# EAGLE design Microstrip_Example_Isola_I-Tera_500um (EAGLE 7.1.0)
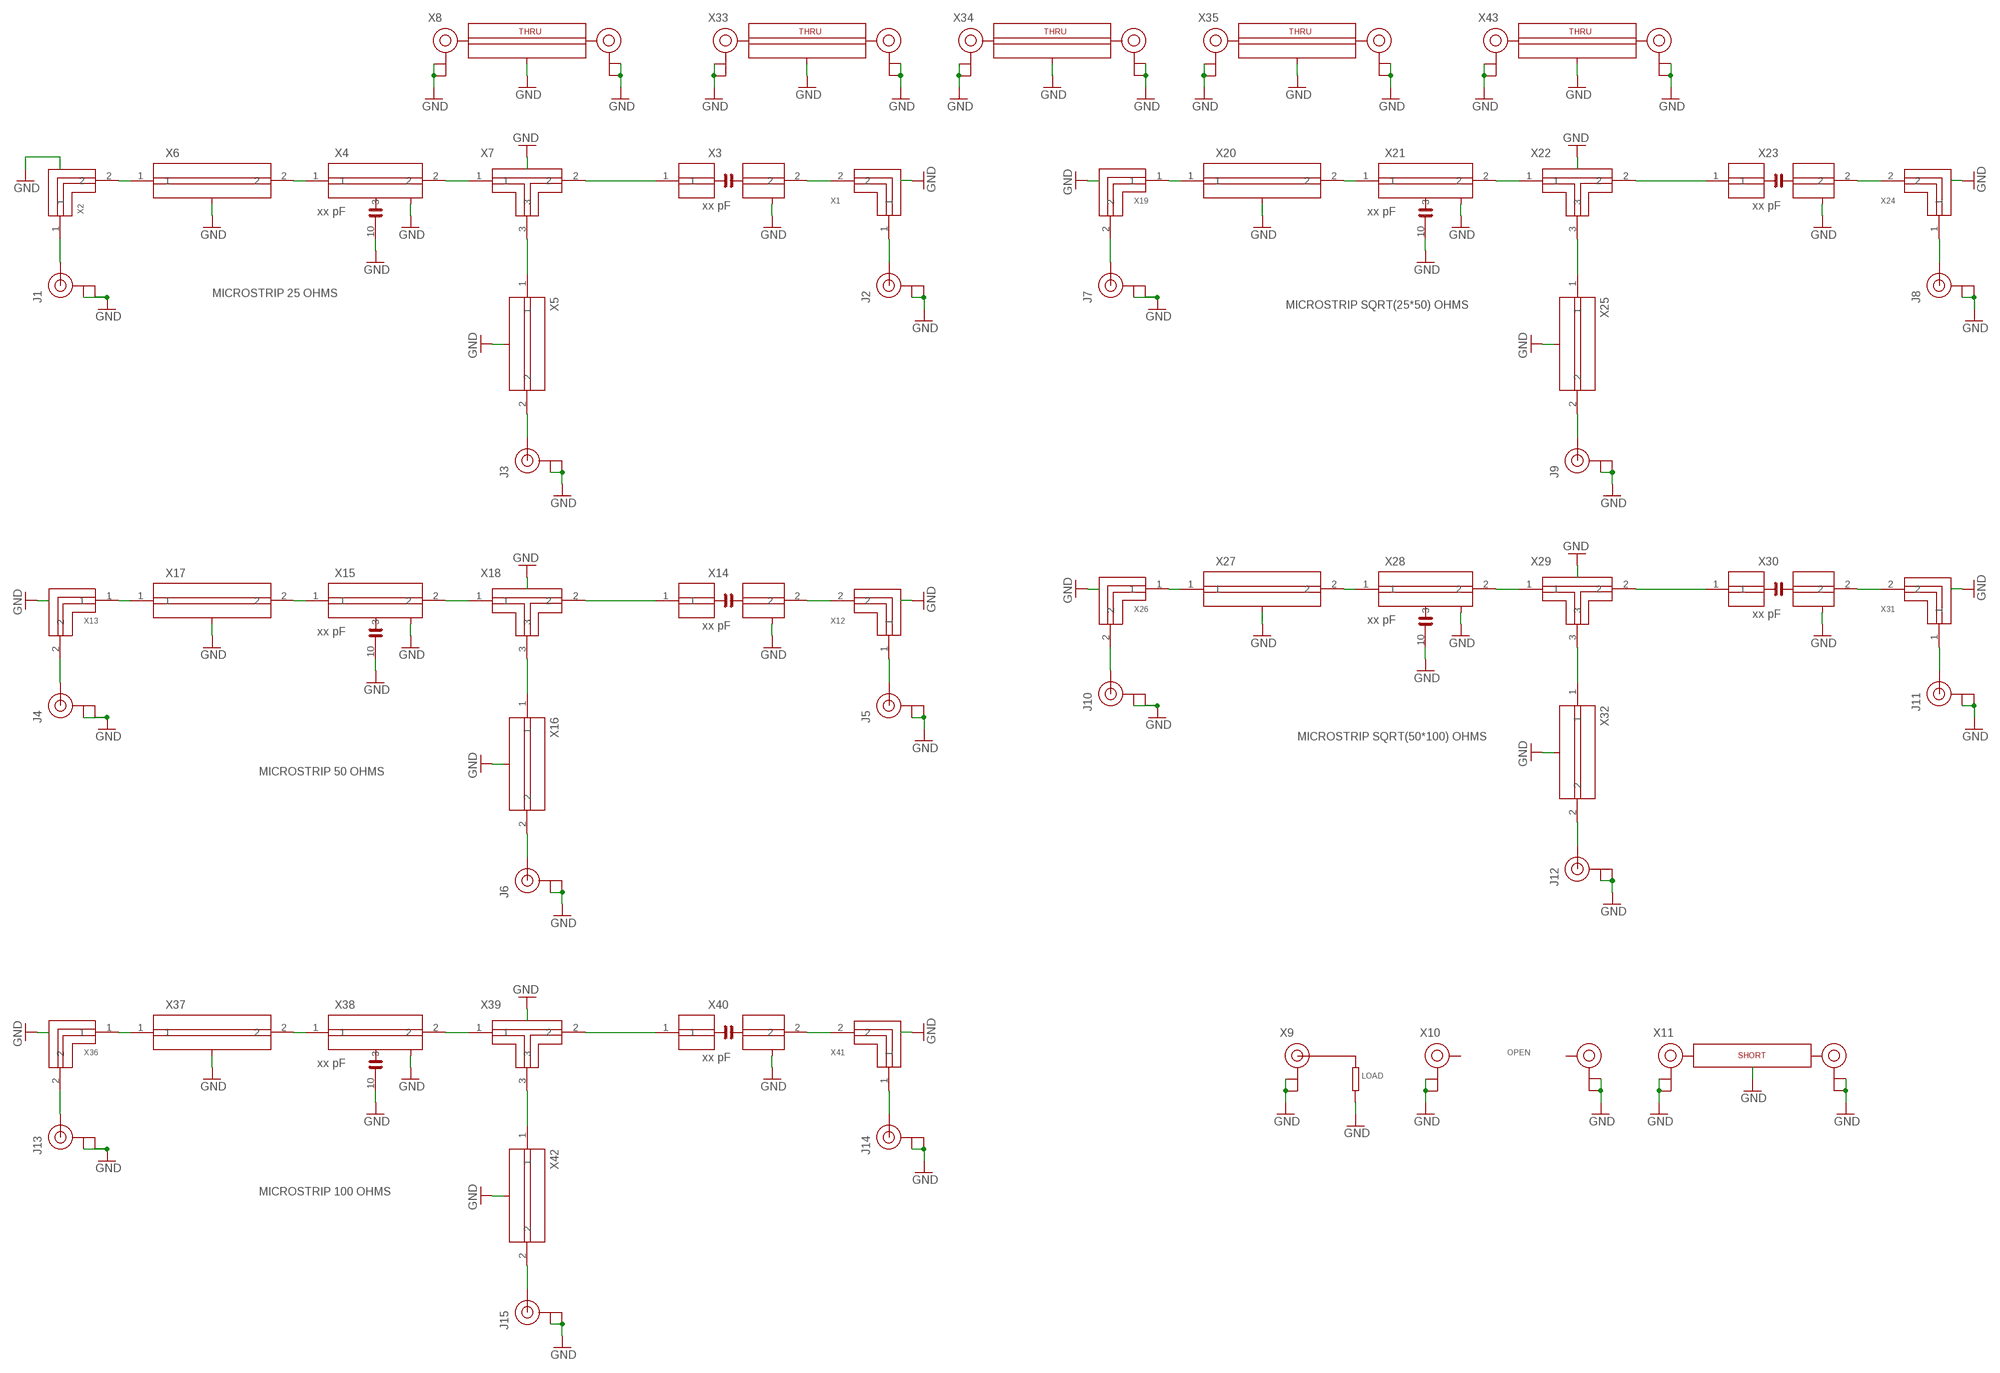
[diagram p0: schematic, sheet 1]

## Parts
J1  U.FL  [U.FL]
J2  U.FL  [U.FL]
J3  U.FL  [U.FL]
J4  U.FL  [U.FL]
J5  U.FL  [U.FL]
J6  U.FL  [U.FL]
J7  U.FL  [U.FL]
J8  U.FL  [U.FL]
J9  U.FL  [U.FL]
J10  U.FL  [U.FL]
J11  U.FL  [U.FL]
J12  U.FL  [U.FL]
J13  U.FL  [U.FL]
J14  U.FL  [U.FL]
J15  U.FL  [U.FL]
X1  CHIPDESIGN_MICROSTRIP_25_OHM_L  [MICROSTRIP_25_OHM_LEFT]
X2  CHIPDESIGN_MICROSTRIP_25_OHM_R  [MICROSTRIP_25_OHM_RIGHT]
X3  xx pF  CHIPDESIGN_MICROSTRIP_25_OHM_SERIES_0402  [MICROSTRIP_25_OHM_0402_SERIES]
X4  xx pF  CHIPDESIGN_MICROSTRIP_25_OHM_SHUNT_0402  [MICROSTRIP_25_OHM_0402_SHUNT]
X5  CHIPDESIGN_MICROSTRIP_25_OHM_TLINE_SHORT  [MICROSTRIP_25_OHM_TLINE_SHORT]
X6  CHIPDESIGN_MICROSTRIP_25_OHM_TLINE_LONG  [MICROSTRIP_25_OHM_TLINE_LONG]
X7  CHIPDESIGN_MICROSTRIP_25_OHM_TJUNCTION  [MICROSTRIP_25_OHM_TEE]
X8  CHIPDESIGN_MICROSTRIP_25_OHM_THRU  [MICROSTRIP_25_OHM_THRU]
X9  LOAD_MICROSTRIP  [LOAD_MICROSTRIP]
X10  OPEN  [OPEN]
X11  SHORT  [SHORT]
X12  CHIPDESIGN_MICROSTRIP_50_OHM_L  [MICROSTRIP_50_OHM_LEFT]
X13  CHIPDESIGN_MICROSTRIP_50_OHM_R  [MICROSTRIP_50_OHM_RIGHT]
X14  xx pF  CHIPDESIGN_MICROSTRIP_50_OHM_SERIES_0402  [MICROSTRIP_50_OHM_0402_SERIES]
X15  xx pF  CHIPDESIGN_MICROSTRIP_50_OHM_SHUNT_0402  [MICROSTRIP_50_OHM_0402_SHUNT]
X16  CHIPDESIGN_MICROSTRIP_50_OHM_TLINE_SHORT  [MICROSTRIP_50_OHM_TLINE_SHORT]
X17  CHIPDESIGN_MICROSTRIP_50_OHM_TLINE_LONG  [MICROSTRIP_50_OHM_TLINE_LONG]
X18  CHIPDESIGN_MICROSTRIP_50_OHM_TJUNCTION  [MICROSTRIP_50_OHM_TEE]
X19  CHIPDESIGN_MICROSTRIP_35_OHM_R  [MICROSTRIP_35_OHM_RIGHT]
X20  CHIPDESIGN_MICROSTRIP_35_OHM_TLINE_LONG  [MICROSTRIP_35_OHM_TLINE_LONG]
X21  xx pF  CHIPDESIGN_MICROSTRIP_35_OHM_SHUNT_0402  [MICROSTRIP_35_OHM_0402_SHUNT]
X22  CHIPDESIGN_MICROSTRIP_35_OHM_TJUNCTION  [MICROSTRIP_35_OHM_TEE]
X23  xx pF  CHIPDESIGN_MICROSTRIP_35_OHM_SERIES_0402  [MICROSTRIP_35_OHM_0402_SERIES]
X24  CHIPDESIGN_MICROSTRIP_35_OHM_L  [MICROSTRIP_35_OHM_LEFT]
X25  CHIPDESIGN_MICROSTRIP_35_OHM_TLINE_SHORT  [MICROSTRIP_35_OHM_TLINE_SHORT]
X26  CHIPDESIGN_MICROSTRIP_70_OHM_R  [MICROSTRIP_70_OHM_RIGHT]
X27  CHIPDESIGN_MICROSTRIP_70_OHM_TLINE_LONG  [MICROSTRIP_70_OHM_TLINE_LONG]
X28  xx pF  CHIPDESIGN_MICROSTRIP_70_OHM_SHUNT_0402  [MICROSTRIP_70_OHM_0402_SHUNT]
X29  CHIPDESIGN_MICROSTRIP_70_OHM_TJUNCTION  [MICROSTRIP_70_OHM_TEE]
X30  xx pF  CHIPDESIGN_MICROSTRIP_70_OHM_SERIES_0402  [MICROSTRIP_70_OHM_0402_SERIES]
X31  CHIPDESIGN_MICROSTRIP_70_OHM_L  [MICROSTRIP_70_OHM_LEFT]
X32  CHIPDESIGN_MICROSTRIP_70_OHM_TLINE_SHORT  [MICROSTRIP_70_OHM_TLINE_SHORT]
X33  CHIPDESIGN_MICROSTRIP_35_OHM_THRU  [MICROSTRIP_35_OHM_THRU]
X34  CHIPDESIGN_MICROSTRIP_50_OHM_THRU  [MICROSTRIP_50_OHM_THRU]
X35  CHIPDESIGN_MICROSTRIP_70_OHM_THRU  [MICROSTRIP_70_OHM_THRU]
X36  CHIPDESIGN_MICROSTRIP_100_OHM_R  [MICROSTRIP_100_OHM_RIGHT]
X37  CHIPDESIGN_MICROSTRIP_100_OHM_TLINE_LONG  [MICROSTRIP_100_OHM_TLINE_LONG]
X38  xx pF  CHIPDESIGN_MICROSTRIP_100_OHM_SHUNT_0402  [MICROSTRIP_100_OHM_0402_SHUNT]
X39  CHIPDESIGN_MICROSTRIP_100_OHM_TJUNCTION  [MICROSTRIP_100_OHM_TEE]
X40  xx pF  CHIPDESIGN_MICROSTRIP_100_OHM_SERIES_0402  [MICROSTRIP_100_OHM_0402_SERIES]
X41  CHIPDESIGN_MICROSTRIP_100_OHM_L  [MICROSTRIP_100_OHM_LEFT]
X42  CHIPDESIGN_MICROSTRIP_100_OHM_TLINE_SHORT  [MICROSTRIP_100_OHM_TLINE_SHORT]
X43  CHIPDESIGN_MICROSTRIP_100_OHM_THRU  [MICROSTRIP_100_OHM_THRU]

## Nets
GND: J1.P$1(GND) J1.P$2(GND) J2.P$1(GND) J2.P$2(GND) J3.P$1(GND) J3.P$2(GND) J4.P$1(GND) J4.P$2(GND) J5.P$1(GND) J5.P$2(GND) J6.P$1(GND) J6.P$2(GND) J7.P$1(GND) J7.P$2(GND) J8.P$1(GND) J8.P$2(GND) J9.P$1(GND) J9.P$2(GND) J10.P$1(GND) J10.P$2(GND) J11.P$1(GND) J11.P$2(GND) J12.P$1(GND) J12.P$2(GND) J13.P$1(GND) J13.P$2(GND) J14.P$1(GND) J14.P$2(GND) J15.P$1(GND) J15.P$2(GND) X1.P$1(GND) X1.P$2(GND) X1.P$3(GND) X1.P$4(GND) X1.P$5(GND) X1.P$6(GND) X1.P$7(GND) X1.P$8(GND) X2.P$1(GND) X2.P$2(GND) X2.P$3(GND) X2.P$4(GND) X2.P$5(GND) X2.P$6(GND) X2.P$7(GND) X2.P$8(GND) X3.P$2(GND) X3.P$3(GND) X3.P$4(GND) X3.P$5(GND) X3.P$6(GND) X3.P$7(GND) X3.P$8(GND) X3.P$9(GND) X3.P$10(GND) X3.P$11(GND) X4.10 X4.P$1(GND) X4.P$2(GND) X4.P$3(GND) X4.P$4(GND) X4.P$5(GND) X4.P$6(GND) X4.P$7(GND) X4.P$8(GND) X4.P$9(GND) X5.P$1(GND) X5.P$2(GND) X5.P$3(GND) X5.P$4(GND) X6.P$1(GND) X6.P$2(GND) X6.P$3(GND) X6.P$4(GND) X6.P$5(GND) X6.P$6(GND) X6.P$7(GND) X6.P$8(GND) X6.P$9(GND) X6.P$10(GND) X7.P$1(GND) X7.P$2(GND) X7.P$3(GND) X7.P$4(GND) X7.P$5(GND) X7.P$6(GND) X7.P$7(GND) X7.P$8(GND) X8.3(GND) X8.4(GND) X8.5(GND) X8.6(GND) X8.7(GND) X8.8(GND) X8.P$1(GND) X8.P$2(GND) X8.P$5(GND) X8.P$6(GND) X8.P$9(GND) X8.P$10(GND) X8.P$11(GND) X8.P$12(GND) X8.P$13(GND) X8.P$14(GND) X8.P$15(GND) X8.P$16(GND) X8.P$17(GND) X8.P$18(GND) X8.P$19(GND) X8.P$20(GND) X9.P$1(GND) X9.P$2(GND) X9.P$6(GND) X9.P$7(GND) X9.P$8(GND) X9.P$9(GND) X9.P$10(GND) X9.P$11(GND) X9.P$12(GND) X10.P$1(GND) X10.P$2(GND) X10.P$5(GND) X10.P$6(GND) X11.P$1(GND) X11.P$2(GND) X11.P$3(GND) X11.P$5(GND) X11.P$6(GND) X11.P$7(GND) X12.P$1(GND) X12.P$2(GND) X12.P$3(GND) X12.P$4(GND) X12.P$5(GND) X12.P$7(GND) X12.P$8(GND) X13.P$1(GND) X13.P$2(GND) X13.P$3(GND) X13.P$4(GND) X13.P$5(GND) X13.P$7(GND) X13.P$8(GND) X14.P$1(GND) X14.P$2(GND) X14.P$3(GND) X14.P$4(GND) X14.P$5(GND) X14.P$6(GND) X14.P$7(GND) X14.P$8(GND) X14.P$9(GND) X14.P$10(GND) X15.10 X15.P$1(GND) X15.P$2(GND) X15.P$3(GND) X15.P$4(GND) X15.P$5(GND) X15.P$6(GND) X15.P$7(GND) X15.P$8(GND) X15.P$9(GND) X16.P$1(GND) X16.P$2(GND) X16.P$3(GND) X16.P$4(GND) X17.P$1(GND) X17.P$2(GND) X17.P$3(GND) X17.P$4(GND) X17.P$5(GND) X17.P$6(GND) X17.P$7(GND) X17.P$8(GND) X17.P$9(GND) X17.P$10(GND) X18.P$1(GND) X18.P$2(GND) X18.P$3(GND) X18.P$4(GND) X18.P$5(GND) X18.P$6(GND) X18.P$7(GND) X19.P$1(GND) X19.P$2(GND) X19.P$3(GND) X19.P$4(GND) X19.P$5(GND) X19.P$6(GND) X19.P$7(GND) X20.P$1(GND) X20.P$2(GND) X20.P$3(GND) X20.P$4(GND) X20.P$5(GND) X20.P$6(GND) X20.P$7(GND) X20.P$8(GND) X20.P$9(GND) X20.P$10(GND) X21.10 X21.P$2(GND) X21.P$3(GND) X21.P$4(GND) X21.P$5(GND) X21.P$6(GND) X21.P$7(GND) X21.P$8(GND) X21.P$9(GND) X21.P$10(GND) X22.P$1(GND) X22.P$2(GND) X22.P$3(GND) X22.P$4(GND) X22.P$5(GND) X22.P$6(GND) X22.P$7(GND) X23.P$2(GND) X23.P$3(GND) X23.P$4(GND) X23.P$5(GND) X23.P$6(GND) X23.P$7(GND) X23.P$8(GND) X23.P$9(GND) X23.P$10(GND) X23.P$11(GND) X24.P$1(GND) X24.P$2(GND) X24.P$3(GND) X24.P$4(GND) X24.P$5(GND) X24.P$6(GND) X24.P$7(GND) X25.P$1(GND) X25.P$2(GND) X25.P$3(GND) X25.P$4(GND) X26.3(GND) X26.4(GND) X26.5(GND) X26.6(GND) X26.7(GND) X26.8(GND) X26.9(GND) X26.10(GND) X27.3(GND) X27.4(GND) X27.5(GND) X27.6(GND) X27.7(GND) X27.8(GND) X27.9(GND) X27.10(GND) X27.11(GND) X27.12(GND) X28.10 X28.P$1(GND) X28.P$2(GND) X28.P$3(GND) X28.P$4(GND) X28.P$5(GND) X28.P$6(GND) X28.P$7(GND) X28.P$8(GND) X28.P$9(GND) X29.P$1(GND) X29.P$2(GND) X29.P$3(GND) X29.P$4(GND) X29.P$5(GND) X29.P$6(GND) X29.P$7(GND) X30.P$2(GND) X30.P$3(GND) X30.P$4(GND) X30.P$5(GND) X30.P$6(GND) X30.P$7(GND) X30.P$8(GND) X30.P$9(GND) X30.P$10(GND) X30.P$11(GND) X31.3(GND) X31.4(GND) X31.5(GND) X31.6(GND) X31.7(GND) X31.8(GND) X31.9(GND) X31.10(GND) X32.P$1(GND) X32.P$2(GND) X32.P$3(GND) X32.P$4(GND) X33.1(GND) X33.2(GND) X33.3(GND) X33.4(GND) X33.5(GND) X33.6(GND) X33.7(GND) X33.8(GND) X33.9(GND) X33.10(GND) X33.11(GND) X33.12(GND) X33.13(GND) X33.14(GND) X33.15(GND) X33.16(GND) X33.17(GND) X33.18(GND) X33.P$1(GND) X33.P$2(GND) X33.P$5(GND) X33.P$6(GND) X34.1(GND) X34.2(GND) X34.3(GND) X34.4(GND) X34.5(GND) X34.6(GND) X34.7(GND) X34.8(GND) X34.9(GND) X34.10(GND) X34.11(GND) X34.12(GND) X34.13(GND) X34.14(GND) X34.15(GND) X34.16(GND) X34.17(GND) X34.18(GND) X34.P$1(GND) X34.P$2(GND) X34.P$5(GND) X34.P$6(GND) X35.1(GND) X35.2(GND) X35.3(GND) X35.4(GND) X35.5(GND) X35.6(GND) X35.7(GND) X35.8(GND) X35.9(GND) X35.10(GND) X35.11(GND) X35.12(GND) X35.13(GND) X35.14(GND) X35.15(GND) X35.16(GND) X35.17(GND) X35.18(GND) X35.P$1(GND) X35.P$2(GND) X35.P$5(GND) X35.P$6(GND) X36.3(GND) X36.4(GND) X36.5(GND) X36.6(GND) X36.7(GND) X36.8(GND) X36.9(GND) X36.10(GND) X37.3(GND) X37.4(GND) X37.5(GND) X37.6(GND) X37.7(GND) X37.8(GND) X37.9(GND) X37.10(GND) X37.11(GND) X37.12(GND) X38.3(GND) X38.4(GND) X38.5(GND) X38.6(GND) X38.7(GND) X38.8(GND) X38.9(GND) X38.10 X38.11(GND) X38.12(GND) X39.4(GND) X39.5(GND) X39.6(GND) X39.7(GND) X39.8(GND) X39.9(GND) X39.10(GND) X40.3(GND) X40.4(GND) X40.5(GND) X40.6(GND) X40.7(GND) X40.8(GND) X40.9(GND) X40.10(GND) X40.11(GND) X40.12(GND) X41.3(GND) X41.4(GND) X41.5(GND) X41.6(GND) X41.7(GND) X41.8(GND) X41.9(GND) X41.10(GND) X42.3(GND) X42.4(GND) X42.5(GND) X42.6(GND) X43.1(GND) X43.2(GND) X43.3(GND) X43.4(GND) X43.5(GND) X43.6(GND) X43.7(GND) X43.8(GND) X43.9(GND) X43.10(GND) X43.11(GND) X43.12(GND) X43.13(GND) X43.14(GND) X43.15(GND) X43.16(GND) X43.17(GND) X43.18(GND) X43.P$1(GND) X43.P$2(GND) X43.P$5(GND) X43.P$6(GND)
N$1: J1.P$3(SIGNAL) X2.1
N$2: X2.2 X6.1
N$3: X4.1 X6.2
N$4: X4.2 X7.1
N$5: X3.1 X7.2
N$6: X5.1 X7.3
N$7: J3.P$3(SIGNAL) X5.2
N$8: X1.2 X3.2
N$9: J2.P$3(SIGNAL) X1.1
N$11: J4.P$3(SIGNAL) X13.2
N$12: X13.1 X17.1
N$13: X15.1 X17.2
N$14: X15.2 X18.1
N$15: X14.1 X18.2
N$16: X16.1 X18.3
N$17: J6.P$3(SIGNAL) X16.2
N$18: X12.2 X14.2
N$19: J5.P$3(SIGNAL) X12.1
N$20: J7.P$3(SIGNAL) X19.2
N$21: X19.1 X20.1
N$22: X20.2 X21.1
N$23: X21.2 X22.1
N$24: X22.2 X23.1
N$25: X22.3 X25.1
N$26: J9.P$3(SIGNAL) X25.2
N$27: X23.2 X24.2
N$28: J8.P$3(SIGNAL) X24.1
N$29: J10.P$3(SIGNAL) X26.2
N$30: X26.1 X27.1
N$31: X27.2 X28.1
N$32: X28.2 X29.1
N$33: X29.2 X30.1
N$34: X29.3 X32.1
N$35: J12.P$3(SIGNAL) X32.2
N$36: X30.2 X31.2
N$37: J11.P$3(SIGNAL) X31.1
N$38: J13.P$3(SIGNAL) X36.2
N$39: X36.1 X37.1
N$40: X37.2 X38.1
N$41: X38.2 X39.1
N$42: X39.2 X40.1
N$43: X39.3 X42.1
N$44: J15.P$3(SIGNAL) X42.2
N$45: X40.2 X41.2
N$46: J14.P$3(SIGNAL) X41.1

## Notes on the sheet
- MICROSTRIP 25 OHMS
- MICROSTRIP SQRT(25*50) OHMS
- MICROSTRIP SQRT(50*100) OHMS
- MICROSTRIP 50 OHMS
- MICROSTRIP 100 OHMS

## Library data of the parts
J1-J15 = GCPW_isola_025:U.FL: SMD antenna connector- WRL-09144; MPN: U.FL-R-SMT-1(10); OC_NEWARK: 50P8856; PROD_ID: CONN-09193
X1 = Chipdesign_Isola_050:CHIPDESIGN_MICROSTRIP_25_OHM_L: Grounded Coplanar Waveguide Line - left; Relative dielectric constant = 3.45; Thickness of dielectric = 0.5mm.; DIELECTRIC: I-TERA-MT-RF; DK: 3.45; OC_NEWARK: unknown; PCB_THICKNESS: 0.5MM; TRACK_THICKNESS: 35um; ZO: 25 ohms
X2 = Chipdesign_Isola_050:CHIPDESIGN_MICROSTRIP_25_OHM_R: Grounded Coplanar Waveguide Line - right; Relative dielectric constant = 3.45; Thickness of dielectric = 0.5mm.; DIELECTRIC: I-TERA-MT-RF; DK: 3.45; PCB_THICKNESS: 0.5mm; TRACK_THICKNESS: 35um; ZO: 25 ohms
X3 = Chipdesign_Isola_050:CHIPDESIGN_MICROSTRIP_25_OHM_SERIES_0402: Grounded Coplanar Waveguide Line - series cap 0402; Relative dielectric constant = 3.45; Thickness of dielectric = 0.5mm.; DIELECTRIC: I-TERA-MT-RF; DK: 3.45; OC_NEWARK: unknown; PCB_THICKNESS: 0.5MM; TRACK_THICKNESS: 35um; ZO: 25 ohms
X4 = Chipdesign_Isola_050:CHIPDESIGN_MICROSTRIP_25_OHM_SHUNT_0402: Grounded Coplanar Waveguide Line - shunt cap 0402; Relative dielectric constant = 3.45; Thickness of dielectric = 0.5mm.; DIELECTRIC: I-TERA-MT-RF; DK: 3.45; OC_NEWARK: unknown; PCB_THICKNESS: 0.5MM; TRACK_THICKNESS: 35um; ZO: 25 ohms
X5 = Chipdesign_Isola_050:CHIPDESIGN_MICROSTRIP_25_OHM_TLINE_SHORT: Grounded Coplanar Waveguide Line - TLINE; Relative dielectric constant = 3.45; Thickness of dielectric = 0.5mm.; DIELECTRIC: I-TERA-MT-RF; DK: 3.45; OC_NEWARK: unknown; PCB_THICKNESS: 0.5mm; TRACK_THICKNESS: 35um; ZO: 25 ohms
X6 = Chipdesign_Isola_050:CHIPDESIGN_MICROSTRIP_25_OHM_TLINE_LONG: Grounded Coplanar Waveguide Line - TLINE, long; Relative dielectric constant = 3.45; Thickness of dielectric = 0.5mm.; DIELECTRIC: I-TERA-MT-RF; DK: 3.45; OC_NEWARK: unknown; PCB_THICKNESS: 0.5mm; TRACK_THICKNESS: 35um; ZO: 25 ohms
X7 = Chipdesign_Isola_050:CHIPDESIGN_MICROSTRIP_25_OHM_TJUNCTION: Grounded Coplanar Waveguide - T JUNCTION, long; Relative dielectric constant = 3.45; Thickness of dielectric = 0.5mm.; DIELECTRIC: I-TERA-MT-RF; DK: 3.45; OC_NEWARK: unknown; PCB_THICKNESS: 0.5MM; TRACK_THICKNESS: 35um; ZO: 25 ohms
X8 = Chipdesign_Isola_050:CHIPDESIGN_MICROSTRIP_25_OHM_THRU: Relative dielectric constant = 3.45; Thickness of dielectric = 0.5mm.; DIELECTRIC: I-TERA-MT-RF; DK: 3.45; OC_NEWARK: unknown; PCB_THICKNESS: 0.5MM; TRACK_THICKNESS: 35um; ZO: 25 ohms
X9 = Chipdesign_Isola_050:LOAD_MICROSTRIP: Relative dielectric constant = 3.45; Thickness of dielectric = 0.5mm.; OC_NEWARK: unknown
X10 = GCPW_isola_025:OPEN; OC_NEWARK: unknown
X11 = GCPW_isola_025:SHORT: Relative dielectric constant = 3.45; Thickness of dielectric = 0.5mm.; OC_NEWARK: unknown
X12 = Chipdesign_Isola_050:CHIPDESIGN_MICROSTRIP_50_OHM_L: Grounded Coplanar Waveguide Line - left; Relative dielectric constant = 3.45; Thickness of dielectric = 0.5mm.; DIELECTRIC: I-TERA-MT-RF; DK: 3.45; OC_NEWARK: unknown; PCB_THICKNESS: 0.5MM; TRACK_THICKNESS: 35um; ZO: 50 ohms
X13 = Chipdesign_Isola_050:CHIPDESIGN_MICROSTRIP_50_OHM_R: Grounded Coplanar Waveguide Line - right; Relative dielectric constant = 3.45; Thickness of dielectric = 0.5mm.; DIELECTRIC: I-TERA-MT-RF; DK: 3.45; OC_NEWARK: unknown; PCB_THICKNESS: 0.5mm; TRACK_THICKNESS: 35um; ZO: 50 ohms
X14 = Chipdesign_Isola_050:CHIPDESIGN_MICROSTRIP_50_OHM_SERIES_0402: Grounded Coplanar Waveguide Line - series cap 0402; Relative dielectric constant = 3.45; Thickness of dielectric = 0.5mm.; DIELECTRIC: I-TERA-MT-RF; DK: 3.45; OC_NEWARK: unknown; PCB_THICKNESS: 0.5MM; TRACK_THICKNESS: 35um; ZO: 50 ohms
X15 = Chipdesign_Isola_050:CHIPDESIGN_MICROSTRIP_50_OHM_SHUNT_0402: Grounded Coplanar Waveguide Line - shunt cap 0402; Relative dielectric constant = 3.45; Thickness of dielectric = 0.5mm.; DIELECTRIC: I-TERA-MT-RF; DK: 3.45; OC_NEWARK: unknown; PCB_THICKNESS: 0.5MM; TRACK_THICKNESS: 35um; ZO: 50 ohms
X16 = Chipdesign_Isola_050:CHIPDESIGN_MICROSTRIP_50_OHM_TLINE_SHORT: Grounded Coplanar Waveguide Line - TLINE; Relative dielectric constant = 3.45; Thickness of dielectric = 0.5mm.; DIELECTRIC: I-TERA-MT-RF; DK: 3.45; OC_NEWARK: unknown; PCB_THICKNESS: 0.5mm; TRACK_THICKNESS: 35um; ZO: 50 ohms
X17 = Chipdesign_Isola_050:CHIPDESIGN_MICROSTRIP_50_OHM_TLINE_LONG: Grounded Coplanar Waveguide Line - TLINE, long; Relative dielectric constant = 3.45; Thickness of dielectric = 0.5mm.; DIELECTRIC: I-TERA-MT-RF; DK: 3.45; OC_NEWARK: unknown; PCB_THICKNESS: 0.5mm; TRACK_THICKNESS: 35um; ZO: 50 ohms
X18 = Chipdesign_Isola_050:CHIPDESIGN_MICROSTRIP_50_OHM_TJUNCTION: Grounded Coplanar Waveguide - T JUNCTION, long; Relative dielectric constant = 3.45; Thickness of dielectric = 0.5mm.; DIELECTRIC: I-TERA-MT-RF; DK: 3.45; OC_NEWARK: unknown; PCB_THICKNESS: 0.5MM; TRACK_THICKNESS: 35um; ZO: 50 ohms
X19 = Chipdesign_Isola_050:CHIPDESIGN_MICROSTRIP_35_OHM_R: Grounded Coplanar Waveguide Line - right; Relative dielectric constant = 3.45; Thickness of dielectric = 0.5mm.; DIELECTRIC: I-TERA-MT-RF; DK: 3.45; OC_NEWARK: unknown; PCB_THICKNESS: 0.5mm; TRACK_THICKNESS: 35um; ZO: sqrt(25*50) ohms
X20 = Chipdesign_Isola_050:CHIPDESIGN_MICROSTRIP_35_OHM_TLINE_LONG: Grounded Coplanar Waveguide Line - TLINE, long; Relative dielectric constant = 3.45; Thickness of dielectric = 0.5mm.; DIELECTRIC: I-TERA-MT-RF; DK: 3.45; OC_NEWARK: unknown; PCB_THICKNESS: 0.5mm; TRACK_THICKNESS: 35um; ZO: sqrt(25*50) ohms
X21 = Chipdesign_Isola_050:CHIPDESIGN_MICROSTRIP_35_OHM_SHUNT_0402: Grounded Coplanar Waveguide Line - shunt cap 0402; Relative dielectric constant = 3.45; Thickness of dielectric = 0.5mm.; DIELECTRIC: I-TERA-MT-RF; DK: 3.45; OC_NEWARK: unknown; PCB_THICKNESS: 0.5MM; TRACK_THICKNESS: 35um; ZO: sqrt(25*50) ohms
X22 = Chipdesign_Isola_050:CHIPDESIGN_MICROSTRIP_35_OHM_TJUNCTION: Grounded Coplanar Waveguide - T JUNCTION, long; Relative dielectric constant = 3.45; Thickness of dielectric = 0.5mm.; DIELECTRIC: I-TERA-MT-RF; DK: 3.45; OC_NEWARK: unknown; PCB_THICKNESS: 0.5MM; TRACK_THICKNESS: 35um; ZO: sqrt(25*50) ohms
X23 = Chipdesign_Isola_050:CHIPDESIGN_MICROSTRIP_35_OHM_SERIES_0402: Grounded Coplanar Waveguide Line - series cap 0402; Relative dielectric constant = 3.45; Thickness of dielectric = 0.5mm.; DIELECTRIC: I-TERA-MT-RF; DK: 3.45; OC_NEWARK: unknown; PCB_THICKNESS: 0.5MM; TRACK_THICKNESS: 35um; ZO: sqrt(25*50) ohms
X24 = Chipdesign_Isola_050:CHIPDESIGN_MICROSTRIP_35_OHM_L: Grounded Coplanar Waveguide Line - left; Relative dielectric constant = 3.45; Thickness of dielectric = 0.5mm.; DIELECTRIC: I-TERA-MT-RF; DK: 3.45; OC_NEWARK: unknown; PCB_THICKNESS: 0.5MM; TRACK_THICKNESS: 35um; ZO: sqrt(25*50) ohms
X25 = Chipdesign_Isola_050:CHIPDESIGN_MICROSTRIP_35_OHM_TLINE_SHORT: Grounded Coplanar Waveguide Line - TLINE; Relative dielectric constant = 3.45; Thickness of dielectric = 0.5mm.; DIELECTRIC: I-TERA-MT-RF; DK: 3.45; OC_NEWARK: unknown; PCB_THICKNESS: 0.5mm; TRACK_THICKNESS: 35um; ZO: sqrt(25*50) ohms
X26 = Chipdesign_Isola_050:CHIPDESIGN_MICROSTRIP_70_OHM_R: Grounded Coplanar Waveguide Line - right; Relative dielectric constant = 3.45; Thickness of dielectric = 0.5mm.; DIELECTRIC: I-TERA-MT-RF; DK: 3.45; OC_NEWARK: unknown; PCB_THICKNESS: 0.5MM; TRACK_THICKNESS: 35um; ZO: sqrt(50*100) ohms
X27 = Chipdesign_Isola_050:CHIPDESIGN_MICROSTRIP_70_OHM_TLINE_LONG: Grounded Coplanar Waveguide Line - TLINE, long; Relative dielectric constant = 3.45; Thickness of dielectric = 0.5mm.; DIELECTRIC: I-TERA-MT-RF; DK: 3.45; OC_NEWARK: unknown; PCB_THICKNESS: 0.5MM; TRACK_THICKNESS: 35um; ZO: sqrt(50*100) ohms
X28 = Chipdesign_Isola_050:CHIPDESIGN_MICROSTRIP_70_OHM_SHUNT_0402: Grounded Coplanar Waveguide Line - shunt cap 0402; Relative dielectric constant = 3.45; Thickness of dielectric = 0.5mm.; DIELECTRIC: I-TERA-MT-RF; DK: 3.45; OC_NEWARK: unknown; PCB_THICKNESS: 0.5MM; TRACK_THICKNESS: 35um; ZO: sqrt(50*100) ohms
X29 = Chipdesign_Isola_050:CHIPDESIGN_MICROSTRIP_70_OHM_TJUNCTION: Grounded Coplanar Waveguide - T JUNCTION, long; Relative dielectric constant = 3.45; Thickness of dielectric = 0.5mm.; DIELECTRIC: I-TERA-MT-RF; DK: 3.45; OC_NEWARK: unknown; PCB_THICKNESS: 0.5MM; TRACK_THICKNESS: 35um; ZO: sqrt(50*100) ohms
X30 = Chipdesign_Isola_050:CHIPDESIGN_MICROSTRIP_70_OHM_SERIES_0402: Grounded Coplanar Waveguide Line - series cap 0402; Relative dielectric constant = 3.45; Thickness of dielectric = 0.5mm.; DIELECTRIC: I-TERA-MT-RF; DK: 3.45; OC_NEWARK: unknown; PCB_THICKNESS: 0.5MM; TRACK_THICKNESS: 35um; ZO: sqrt(50*100) ohms
X31 = Chipdesign_Isola_050:CHIPDESIGN_MICROSTRIP_70_OHM_L: Grounded Coplanar Waveguide Line - left; Relative dielectric constant = 3.45; Thickness of dielectric = 0.5mm.; DIELECTRIC: I-TERA-MT-RF; DK: 3.45; OC_NEWARK: unknown; PCB_THICKNESS: 0.5MM; TRACK_THICKNESS: 35um; ZO: sqrt(50*100) ohms
X32 = Chipdesign_Isola_050:CHIPDESIGN_MICROSTRIP_70_OHM_TLINE_SHORT: Grounded Coplanar Waveguide Line - TLINE; Relative dielectric constant = 3.45; Thickness of dielectric = 0.5mm.; DIELECTRIC: I-TERA-MT-RF; DK: 3.45; OC_NEWARK: unknown; PCB_THICKNESS: 0.5mm; TRACK_THICKNESS: 35um; ZO: sqrt(50*100) ohms
X33 = Chipdesign_Isola_050:CHIPDESIGN_MICROSTRIP_35_OHM_THRU: Relative dielectric constant = 3.45; Thickness of dielectric = 0.5mm.; DIELECTRIC: I-TERA-MT-RF; DK: 3.45; OC_NEWARK: unknown; PCB_THICKNESS: 0.5mm; TRACK_THICKNESS: 35um; ZO: sqrt(25*50) ohms
X34 = Chipdesign_Isola_050:CHIPDESIGN_MICROSTRIP_50_OHM_THRU: Relative dielectric constant = 3.45; Thickness of dielectric = 0.5mm.; DIELECTRIC: I-TERA-MT-RF; DK: 3.45; OC_NEWARK: unknown; PCB_THICKNESS: 0.5MM; TRACK_THICKNESS: 35um; ZO: 50 ohms
X35 = Chipdesign_Isola_050:CHIPDESIGN_MICROSTRIP_70_OHM_THRU: Relative dielectric constant = 3.45; Thickness of dielectric = 0.5mm.; DIELECTRIC: I-TERA-MT-RF; DK: 3.45; OC_NEWARK: unknown; PCB_THICKNESS: 0.5MM; TRACK_THICKNESS: 35um; ZO: sqrt(50*100) ohms
X36 = Chipdesign_Isola_050:CHIPDESIGN_MICROSTRIP_100_OHM_R: Grounded Coplanar Waveguide Line - right; Relative dielectric constant = 3.45; Thickness of dielectric = 0.5mm.; DIELECTRIC: I-TERA-MT-RF; DK: 3.45; OC_NEWARK: unknown; PCB_THICKNESS: 0.5MM; TRACK_THICKNESS: 35um; ZO: 100 ohms
X37 = Chipdesign_Isola_050:CHIPDESIGN_MICROSTRIP_100_OHM_TLINE_LONG: Grounded Coplanar Waveguide Line - TLINE, long; Relative dielectric constant = 3.45; Thickness of dielectric = 0.5mm.; DIELECTRIC: I-TERA-MT-RF; DK: 3.45; OC_NEWARK: unknown; PCB_THICKNESS: 0.5MM; TRACK_THICKNESS: 35um; ZO: 100 ohms
X38 = Chipdesign_Isola_050:CHIPDESIGN_MICROSTRIP_100_OHM_SHUNT_0402: Grounded Coplanar Waveguide Line - shunt cap 0402; Relative dielectric constant = 3.45; Thickness of dielectric = 0.5mm.; DIELECTRIC: I-TERA-MT-RF; DK: 3.45; OC_NEWARK: unknown; PCB_THICKNESS: 0.5MM; TRACK_THICKNESS: 35um; ZO: 100 ohms
X39 = Chipdesign_Isola_050:CHIPDESIGN_MICROSTRIP_100_OHM_TJUNCTION: Grounded Coplanar Waveguide - T JUNCTION, long; Relative dielectric constant = 3.45; Thickness of dielectric = 0.5mm.; DIELECTRIC: I-TERA-MT-RF; DK: 3.45; OC_NEWARK: unknown; PCB_THICKNESS: 0.5MM; TRACK_THICKNESS: 35um; ZO: 100 ohms
X40 = Chipdesign_Isola_050:CHIPDESIGN_MICROSTRIP_100_OHM_SERIES_0402: Grounded Coplanar Waveguide Line - series cap 0402; Relative dielectric constant = 3.45; Thickness of dielectric = 0.5mm.; DIELECTRIC: I-TERA-MT-RF; DK: 3.45; OC_NEWARK: unknown; PCB_THICKNESS: 0.5MM; TRACK_THICKNESS: 35um; ZO: 100 ohms
X41 = Chipdesign_Isola_050:CHIPDESIGN_MICROSTRIP_100_OHM_L: Grounded Coplanar Waveguide Line - left; Relative dielectric constant = 3.45; Thickness of dielectric = 0.5mm.; DIELECTRIC: I-TERA-MT-RF; DK: 3.45; OC_NEWARK: unknown; PCB_THICKNESS: 0.5MM; TRACK_THICKNESS: 35um; ZO: 100 ohms
X42 = Chipdesign_Isola_050:CHIPDESIGN_MICROSTRIP_100_OHM_TLINE_SHORT: Grounded Coplanar Waveguide Line - TLINE; Relative dielectric constant = 3.45; Thickness of dielectric = 0.5mm.; DIELECTRIC: I-TERA-MT-RF; DK: 3.45; OC_NEWARK: unknown; PCB_THICKNESS: 0.5MM; TRACK_THICKNESS: 35um; ZO: 100 ohms
X43 = Chipdesign_Isola_050:CHIPDESIGN_MICROSTRIP_100_OHM_THRU: Relative dielectric constant = 3.45; Thickness of dielectric = 0.5mm.; DIELECTRIC: I-TERA-MT-RF; DK: 3.45; OC_NEWARK: unknown; PCB_THICKNESS: 0.5MM; TRACK_THICKNESS: 35um; ZO: 100 ohms

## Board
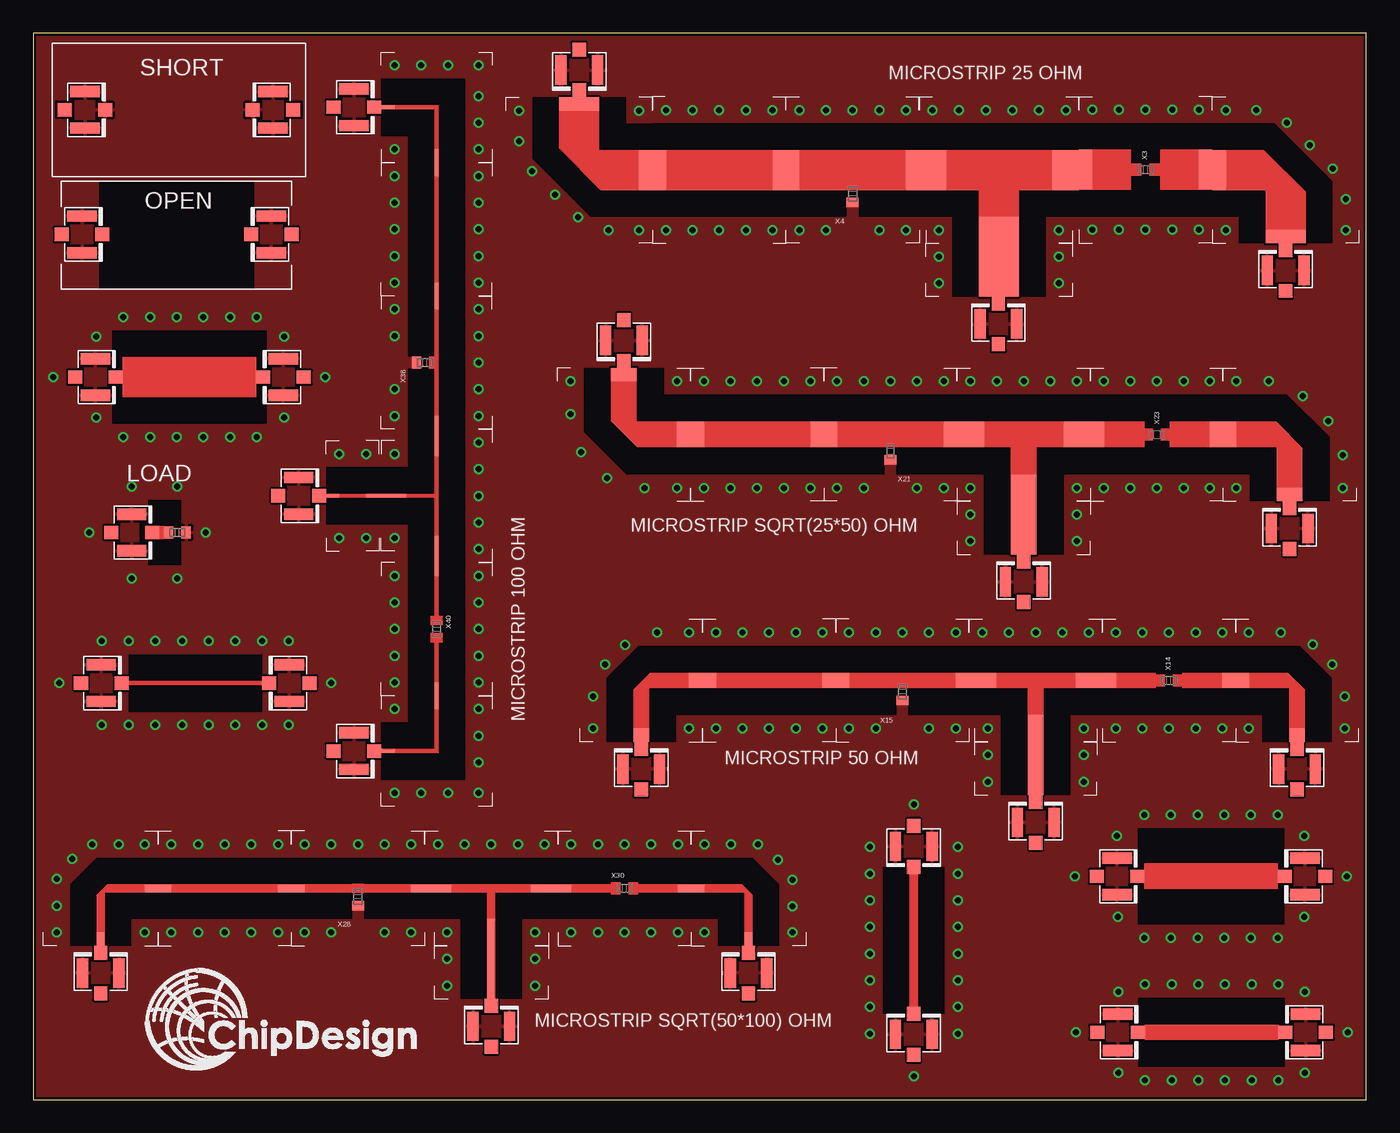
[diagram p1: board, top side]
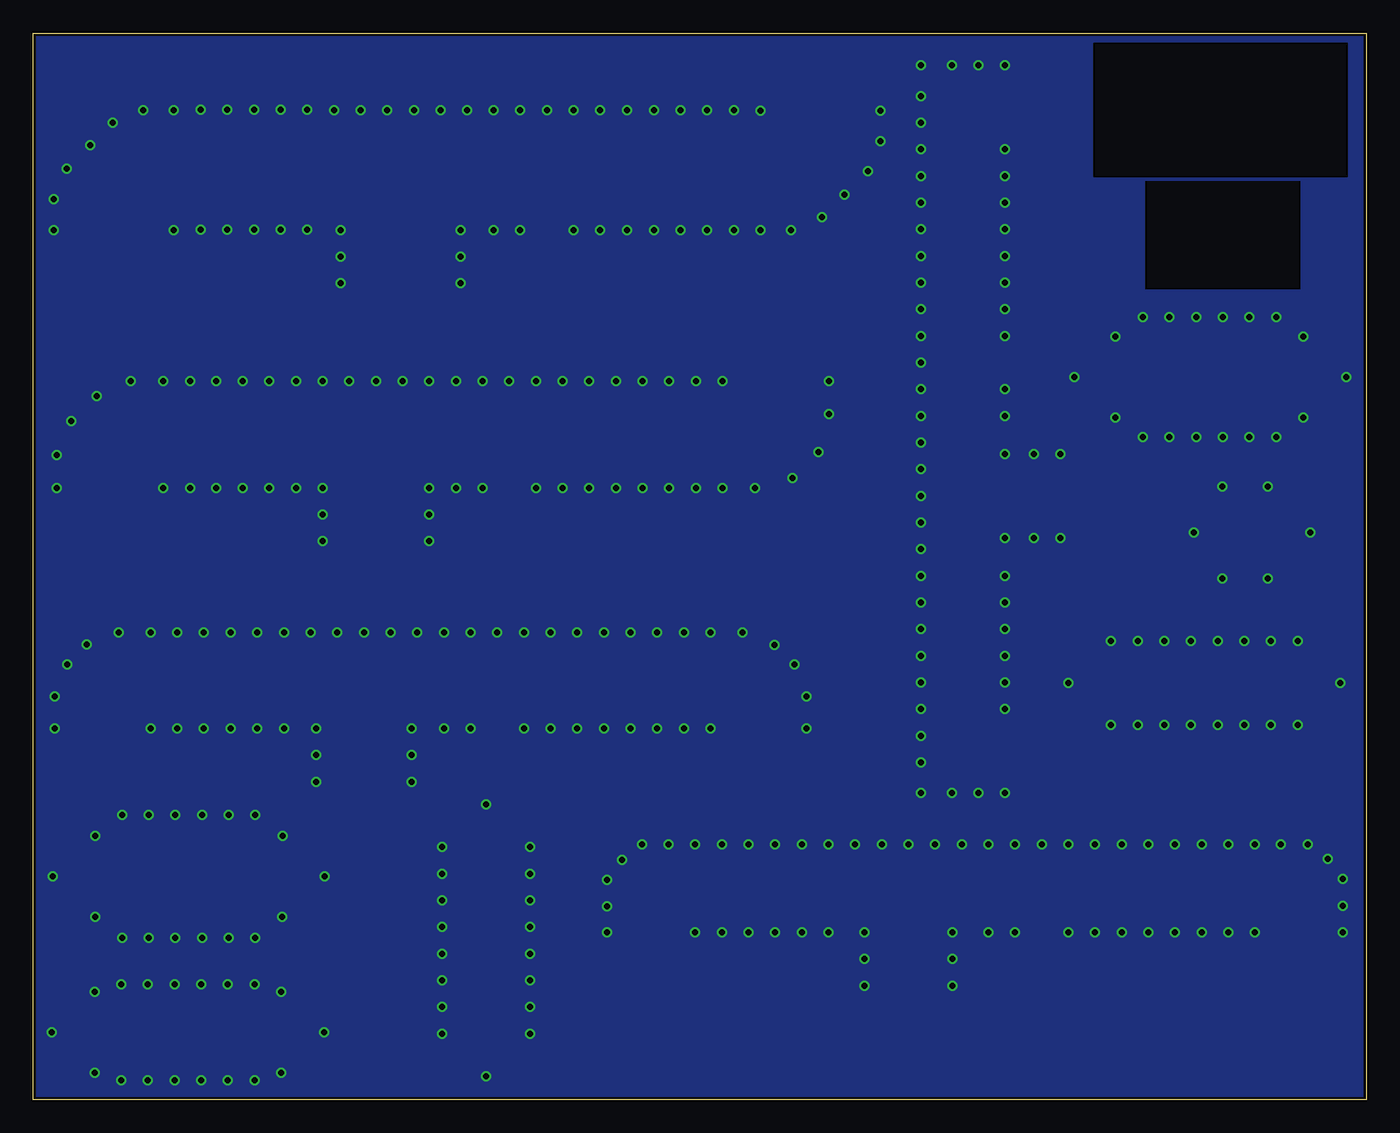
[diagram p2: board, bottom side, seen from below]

Size 100 x 80 mm. Coordinates in mm from the lower left corner, seen from the top.
Outline: 0,0 100,0 100,80 0,80 0,0
Copper layers (1*16): Top 0.035mm / dielectric 1.5mm / Bottom 0.035mm
Design rules "Eagle-DRU - 1506 - LeitOn - 01 and 02 layers - STANDARD": minimum track width 0.15mm, minimum drill 0.3mm, track to track 0.15mm, track to pad 0.15mm, pad to pad 0.15mm, via to via 0.15mm, smd to smd 0.15mm, copper to edge 0.2mm, drill to drill 0.25mm, minimum pad ring 0.15mm, minimum via ring 0.15mm, stop-mask expansion 0.05mm, vias tented up to drill 0mil, thermal gap 0.2mm

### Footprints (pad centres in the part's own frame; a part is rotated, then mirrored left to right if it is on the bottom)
U.FL = smd 2.2 x 0.85: P$1 0,1.375; P$2 0,-1.375 | smd 1.05 x 1: P$3 1.525,0; P$4 -1.525,0
MICROSTRIP_25_OHM_LEFT = smd 3 x 1: 1 5,-5 | smd 1 x 3: 2 0,0 | drill 0.45: P$1 0.5,-4.5; P$2 0.5,4.5; P$3 2.8,4.5; P$4 5.1,3.55; P$5 6.8,1.85; P$6 8.55,0.1; P$7 9.5,-2.2; P$8 9.5,-4.5
MICROSTRIP_25_OHM_RIGHT = smd 1 x 3: 1 0,0 | smd 3 x 1: 2 -4.95,-5 | drill 0.45: P$1 -0.5,-4.5; P$2 -9.45,-4.5; P$3 -9.45,-2.2; P$4 -8.5,0.1; P$5 -6.8,1.8; P$6 -5.05,3.55; P$7 -2.8,4.5; P$8 -0.5,4.5
MICROSTRIP_25_OHM_0402_SERIES = smd 1 x 3: 1 -4.5,0; 2 4.5,0 | drill 0.45: P$2 -4,4.5; P$3 -2,4.5; P$4 0,4.5; P$5 2,4.5; P$6 4,4.5; P$7 -4,-4.5; P$8 -2,-4.5; P$9 0,-4.5; P$10 2,-4.5; P$11 4,-4.5
MICROSTRIP_25_OHM_0402_SHUNT = smd 1 x 3: 1 -4.5,1.8; 2 4.5,1.8 | smd 0.9 x 0.7: 10 0,-0.65 | drill 0.45: P$1 -4,-2.7; P$2 -4,6.3; P$3 -2,6.3; P$4 0,6.3; P$5 2,6.3; P$6 4,6.3; P$7 -2,-2.7; P$8 2,-2.7; P$9 4,-2.7
MICROSTRIP_25_OHM_TLINE_SHORT = smd 2 x 3: 1 0.5,0; 2 2.5,0 | drill 0.45: P$1 0.5,4.5; P$2 2.5,4.5; P$3 0.5,-4.5; P$4 2.5,-4.5
MICROSTRIP_25_OHM_TLINE_LONG = smd 1 x 3: 1 0,0; 2 9,0 | drill 0.45: P$1 0.5,-4.5; P$2 0.5,4.5; P$3 2.5,4.5; P$4 4.5,4.5; P$5 6.5,4.5; P$6 8.5,4.5; P$7 2.5,-4.5; P$8 4.5,-4.5; P$9 6.5,-4.5; P$10 8.5,-4.5
MICROSTRIP_25_OHM_TEE = smd 2 x 3: 1 -5,4.5; 2 5,4.5 | smd 3 x 2: 3 0,0 | drill 0.45: P$1 -5,9; P$2 -3,9; P$3 -1,9; P$4 1,9; P$5 3,9; P$6 5,9; P$7 4.5,0; P$8 -4.5,0
MICROSTRIP_25_OHM_THRU = drill 0.45: 3 -2.5,3.05; 4 -5.7,0; 5 -2.5,-3.05; 6 11.6,-3.05; 7 14.7,0; 8 11.6,3.05; P$9 -0.45,4.5; P$10 1.55,4.5; P$11 3.55,4.5; P$12 5.55,4.5; P$13 7.55,4.5; P$14 9.55,4.5; P$15 -0.45,-4.5; P$16 1.55,-4.5; P$17 3.55,-4.5; P$18 5.55,-4.5; P$19 7.55,-4.5; P$20 9.55,-4.5 | smd 2.2 x 0.85: P$1 -2.55,1.375; P$2 -2.55,-1.375; P$5 11.55,-1.375; P$6 11.55,1.375 | smd 1.05 x 1: P$3 -1.025,0; P$4 -4.075,0; P$7 10.025,0; P$8 13.075,0
LOAD_MICROSTRIP = smd 2.2 x 0.85: P$1 -3.425,1.375; P$2 -3.425,-1.375 | smd 1.05 x 1: P$3 -1.9,0; P$4 -4.95,0 | smd 0.7 x 0.9: P$5 -0.65,0; P$6 0.65,0 | drill 0.45: P$7 2.125,0; P$8 0,3.45; P$9 -3.425,3.45; P$10 -6.6,0; P$11 -3.425,-3.45; P$12 0,-3.45
OPEN = smd 2.2 x 0.85: P$1 -1.525,1.375; P$2 -1.525,-1.375; P$5 12.675,-1.375; P$6 12.675,1.375 | smd 1.05 x 1: P$3 0,0; P$4 -3.05,0; P$7 11.15,0; P$8 14.2,0
SHORT = smd 2.2 x 0.85: P$1 -1.55,1.375; P$2 -1.55,-1.375; P$5 12.55,-1.375; P$6 12.55,1.375 | smd 1.05 x 1: P$3 -0.025,0; P$4 -3.075,0; P$7 11.025,0; P$8 14.075,0
MICROSTRIP_50_OHM_LEFT = smd 1.15 x 1: 1 4.1,-4.1 | smd 1 x 1.15: 2 0,0 | drill 0.45: P$1 0.5,3.6; P$2 2.9,3.6; P$3 0.5,-3.6; P$4 7.7,-3.6; P$5 7.7,-1.2; P$7 6.75,1.2; P$8 5.3,2.7
MICROSTRIP_50_OHM_RIGHT = smd 1 x 1.15: 1 0,0 | smd 1.15 x 1: 2 -4.1,-4.1 | drill 0.45: P$1 -7.7,-3.6; P$2 -7.7,-1.2; P$3 -0.5,-3.6; P$4 -0.5,3.6; P$5 -2.9,3.6; P$7 -5.3,2.65; P$8 -6.8,1.2
MICROSTRIP_50_OHM_0402_SERIES = smd 1 x 1.15: 1 -4.5,0; 2 4.5,0 | drill 0.45: P$1 -4,3.6; P$2 -2,3.6; P$3 0,3.6; P$4 2,3.6; P$5 4,3.6; P$6 -4,-3.6; P$7 -2,-3.6; P$8 0,-3.6; P$9 2,-3.6; P$10 4,-3.6
MICROSTRIP_50_OHM_0402_SHUNT = smd 1 x 1.15: 1 -4.5,0.85; 2 4.5,0.85 | smd 0.9 x 0.7: 10 0,-0.65 | drill 0.45: P$1 -4,4.45; P$2 -2,4.45; P$3 0,4.45; P$4 2,4.45; P$5 4,4.45; P$6 -4,-2.75; P$7 -2,-2.75; P$8 4,-2.75; P$9 2,-2.75
MICROSTRIP_50_OHM_TLINE_SHORT = smd 2 x 1.15: 1 0.5,0; 2 2.5,0 | drill 0.45: P$1 0.5,3.6; P$2 2.5,3.6; P$3 0.5,-3.6; P$4 2.5,-3.6
MICROSTRIP_50_OHM_TLINE_LONG = smd 1 x 1.15: 1 0,0; 2 9,0 | drill 0.45: P$1 0.5,3.6; P$2 8.5,3.6; P$3 0.5,-3.6; P$4 8.5,-3.6; P$5 2.5,3.6; P$6 4.5,3.6; P$7 6.5,3.6; P$8 2.5,-3.6; P$9 4.5,-3.6; P$10 6.5,-3.6
MICROSTRIP_50_OHM_TEE = smd 2 x 1.15: 1 -4,3.6; 2 4,3.6 | smd 1.15 x 2: 3 0,0 | drill 0.45: P$1 -4,7.2; P$2 4,7.2; P$3 -2,7.2; P$4 0,7.2; P$5 -3.6,0; P$6 2,7.2; P$7 3.6,0
MICROSTRIP_35_OHM_RIGHT = smd 1.92 x 1: 1 -4.5,-4.5 | smd 1 x 1.92: 2 0,0 | drill 0.45: P$1 -0.5,4; P$2 -2.95,4; P$3 -8.5,-4; P$4 -8.5,-1.55; P$5 -7.75,1.25; P$6 -5.8,3.2; P$7 -0.5,-4
MICROSTRIP_35_OHM_TLINE_LONG = smd 1 x 1.92: 1 0,0; 2 9,0 | drill 0.45: P$1 0.5,4; P$2 2.5,4; P$3 4.5,4; P$4 6.5,4; P$5 8.5,4; P$6 0.5,-4; P$7 2.5,-4; P$8 4.5,-4; P$9 6.5,-4; P$10 8.5,-4
MICROSTRIP_35_OHM_0402_SHUNT = smd 1 x 1.92: 1 -4.5,1.25; 2 4.5,1.25 | smd 0.9 x 0.7: 10 0,-0.65 | drill 0.45: P$2 -4,5.25; P$3 -2,5.25; P$4 0,5.25; P$5 2,5.25; P$6 4,5.25; P$7 -4,-2.75; P$8 -2,-2.75; P$9 2,-2.75; P$10 4,-2.75
MICROSTRIP_35_OHM_TEE = smd 2 x 1.92: 1 -4,4; 2 4,4 | smd 1.92 x 2: 3 0,0 | drill 0.45: P$1 -4,8; P$2 -2,8; P$3 0,8; P$4 2,8; P$5 4,8; P$6 4,0; P$7 -4,0
MICROSTRIP_35_OHM_0402_SERIES = smd 1 x 1.92: 1 -4.5,0; 2 4.45,0 | drill 0.45: P$2 -4,4; P$3 -2,4; P$4 0,4; P$5 2,4; P$6 3.95,4; P$7 -4,-4; P$8 -2,-4; P$9 0,-4; P$10 2,-4; P$11 3.95,-4
MICROSTRIP_35_OHM_LEFT = smd 1.92 x 1: 1 4.5,-4.5 | smd 1 x 1.92: 2 0,0 | drill 0.45: P$1 0.5,4; P$2 2.95,4; P$3 5.5,2.9; P$4 7.4,1; P$5 8.5,-1.55; P$6 8.5,-4; P$7 0.5,-4
MICROSTRIP_35_OHM_TLINE_SHORT = smd 2 x 1.92: 1 0.5,0; 2 2.5,0 | drill 0.45: P$1 0.5,4; P$2 2.5,4; P$3 0.5,-4; P$4 2.5,-4
MICROSTRIP_70_OHM_RIGHT = smd 1 x 0.62: 1 0,0 | smd 0.62 x 1: 2 -3.8,-3.8 | drill 0.45: 3 -0.5,-3.3; 4 -7.1,-1.3; 5 -7.1,-3.3; 6 -7.1,0.7; 7 -5.95,2.2; 8 -4.45,3.3; 9 -2.45,3.3; 10 -0.5,3.3
MICROSTRIP_70_OHM_TLINE_LONG = smd 1 x 0.62: 1 0,0; 2 9,0 | drill 0.45: 3 0.5,3.3; 4 2.5,3.3; 5 4.5,3.3; 6 6.5,3.3; 7 8.5,3.3; 8 8.5,-3.3; 9 6.5,-3.3; 10 4.5,-3.3; 11 2.5,-3.3; 12 0.5,-3.3
MICROSTRIP_70_OHM_0402_SHUNT = smd 1 x 0.62: 1 -4.5,0.65; 2 4.5,0.65 | smd 0.9 x 0.7: 10 0,-0.65 | drill 0.45: P$1 -4,3.95; P$2 -2,3.95; P$3 0,3.95; P$4 2,3.95; P$5 4,3.95; P$6 -4,-2.65; P$7 -2,-2.65; P$8 2,-2.65; P$9 4,-2.65
MICROSTRIP_70_OHM_TEE = smd 2 x 0.62: 1 -4,3.3; 2 4,3.3 | smd 0.62 x 2: 3 0,0 | drill 0.45: P$1 -4,6.6; P$2 -2,6.6; P$3 0,6.6; P$4 2,6.6; P$5 4,6.6; P$6 3.3,0; P$7 -3.3,0
MICROSTRIP_70_OHM_0402_SERIES = smd 1 x 0.62: 1 -4.5,0; 2 4.5,0 | drill 0.45: P$2 -4,3.3; P$3 -2,3.3; P$4 0,3.3; P$5 2,3.3; P$6 4,3.3; P$7 -4,-3.3; P$8 -2,-3.3; P$9 0,-3.3; P$10 2,-3.3; P$11 4,-3.3
MICROSTRIP_70_OHM_LEFT = smd 0.62 x 1: 1 3.8,-3.8 | smd 1 x 0.62: 2 0,0 | drill 0.45: 3 0.5,-3.3; 4 2.5,3.3; 5 0.5,3.3; 6 4.5,3.3; 7 6,2.15; 8 7.1,0.65; 9 7.1,-1.35; 10 7.1,-3.3
MICROSTRIP_70_OHM_TLINE_SHORT = smd 2 x 0.62: 1 0.5,0; 2 2.5,0 | drill 0.45: P$1 0.5,3.3; P$2 2.5,3.3; P$3 0.5,-3.3; P$4 2.5,-3.3
MICROSTRIP_35_OHM_THRU = drill 0.45: 1 -0.5,4.6; 2 1.5,4.6; 3 -2.5,3.05; 4 -5.7,0; 5 -2.5,-3.05; 6 11.55,-3.05; 7 14.7,0; 8 11.5,3.05; 9 3.5,4.6; 10 5.5,4.6; 11 7.5,4.6; 12 9.5,4.6; 13 -0.5,-4.6; 14 1.5,-4.6; 15 3.5,-4.6; 16 5.5,-4.6; 17 7.5,-4.6; 18 9.5,-4.6 | smd 2.2 x 0.85: P$1 -2.55,1.375; P$2 -2.55,-1.375; P$5 11.55,-1.375; P$6 11.55,1.375 | smd 1.05 x 1: P$3 -1.025,0; P$4 -4.075,0; P$7 10.025,0; P$8 13.075,0
MICROSTRIP_50_OHM_THRU = drill 0.45: 1 -0.5,3.6; 2 1.5,3.6; 3 -2.5,3.05; 4 -5.7,0; 5 -2.5,-3.05; 6 11.5,-3.05; 7 14.7,0; 8 11.5,3.05; 9 3.5,3.6; 10 5.5,3.6; 11 7.5,3.6; 12 9.5,3.6; 13 -0.5,-3.6; 14 1.5,-3.6; 15 3.5,-3.6; 16 5.5,-3.6; 17 7.5,-3.6; 18 9.5,-3.6 | smd 2.2 x 0.85: P$1 -2.55,1.375; P$2 -2.55,-1.375; P$5 11.55,-1.375; P$6 11.55,1.375 | smd 1.05 x 1: P$3 -1.025,0; P$4 -4.075,0; P$7 10.025,0; P$8 13.075,0
MICROSTRIP_70_OHM_THRU = drill 0.45: 1 -0.5,3.3; 2 1.5,3.3; 3 -2.5,3.3; 4 -5.7,0; 5 -2.5,-3.3; 6 11.5,-3.3; 7 14.7,0; 8 11.5,3.3; 9 3.5,3.3; 10 5.5,3.3; 11 7.5,3.3; 12 9.5,3.3; 13 -0.5,-3.3; 14 1.5,-3.3; 15 3.5,-3.3; 16 5.5,-3.3; 17 7.5,-3.3; 18 9.5,-3.3 | smd 2.2 x 0.85: P$1 -2.55,1.375; P$2 -2.55,-1.375; P$5 11.55,-1.375; P$6 11.55,1.375 | smd 1.05 x 1: P$3 -1.025,0; P$4 -4.075,0; P$7 10.025,0; P$8 13.075,0
MICROSTRIP_100_OHM_RIGHT = smd 1 x 0.288: 1 0,0 | smd 0.288 x 1: 2 -3.65,-3.65 | drill 0.45: 3 -0.5,-3.15; 4 -6.8,3.15; 5 -4.5,3.15; 6 -6.8,-3.15; 7 -6.8,-1.15; 8 -6.8,0.85; 9 -2.5,3.15; 10 -0.5,3.15
MICROSTRIP_100_OHM_TLINE_LONG = smd 1 x 0.288: 1 0,0; 2 9,0 | drill 0.45: 3 0.5,3.15; 4 2.5,3.15; 5 0.5,-3.15; 6 2.5,-3.15; 7 4.5,3.15; 8 4.5,-3.15; 9 6.5,-3.15; 10 6.5,3.15; 11 8.5,3.15; 12 8.5,-3.15
MICROSTRIP_100_OHM_0402_SHUNT = smd 1 x 0.288: 1 -4.5,0.85; 2 4.5,0.85 | drill 0.45: 3 -4,4; 4 -2,4; 5 0,4; 6 2,4; 7 4,4; 8 -4,-2.3; 9 -2,-2.3; 11 2,-2.3; 12 4,-2.3 | smd 0.9 x 0.7: 10 0,-0.65
MICROSTRIP_100_OHM_TEE = smd 2 x 0.288: 1 -4,3.3; 2 4,3.3 | smd 0.288 x 2: 3 0,0 | drill 0.45: 4 -3.15,0.15; 5 3.15,0.15; 6 4,6.45; 7 2,6.45; 8 0,6.45; 9 -2,6.45; 10 -4,6.45
MICROSTRIP_100_OHM_0402_SERIES = smd 1 x 0.288: 1 -4.5,0; 2 4.5,0 | drill 0.45: 3 -4,3.15; 4 -2,3.15; 5 -4,-3.15; 6 -2,-3.15; 7 2,3.15; 8 2,-3.15; 9 4,-3.15; 10 4,3.15; 11 0,3.15; 12 0,-3.15
MICROSTRIP_100_OHM_LEFT = smd 0.288 x 1: 1 3.65,-3.65 | smd 1 x 0.288: 2 0,0 | drill 0.45: 3 0.5,-3.15; 4 6.8,3.15; 5 6.8,0.85; 6 0.5,3.15; 7 2.5,3.15; 8 4.5,3.15; 9 6.8,-1.15; 10 6.8,-3.15
MICROSTRIP_100_OHM_TLINE_SHORT = smd 1 x 0.288: 1 0,0; 2 3,0 | drill 0.45: 3 0.5,3.15; 4 2.5,3.15; 5 0.5,-3.15; 6 2.5,-3.15
MICROSTRIP_100_OHM_THRU = drill 0.45: 1 -5.7,0; 2 -2.5,3.15; 3 -0.5,3.15; 4 1.5,3.15; 5 3.5,3.15; 6 5.5,3.15; 7 7.5,3.15; 8 9.5,3.15; 9 11.5,3.15; 10 14.7,0; 11 11.5,-3.15; 12 9.5,-3.15; 13 7.5,-3.15; 14 5.5,-3.15; 15 3.5,-3.15; 16 1.5,-3.15; 17 -0.5,-3.15; 18 -2.5,-3.15 | smd 2.2 x 0.85: P$1 -2.55,1.375; P$2 -2.55,-1.375; P$5 11.55,-1.375; P$6 11.55,1.375 | smd 1.05 x 1: P$3 -1.025,0; P$4 -4.075,0; P$7 10.025,0; P$8 13.075,0

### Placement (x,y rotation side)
J1  40.95,77.25 270 top
J2  93.95,62.2 90 top
J3  72.4,58.2 90 top
J4  45.6,24.8 90 top
J5  94.8,24.8 90 top
J6  75.2,20.8 90 top
J7  44.3,56.95 270 top
J8  94.25,42.85 90 top
J9  74.3,38.85 90 top
J10  5.05,9.5 90 top
J11  53.65,9.5 90 top
J12  34.35,5.5 90 top
J13  24.05,74.45 0 top
J14  24.05,26.15 0 top
J15  19.9,45.3 0 top
X1  88.95,69.75 0 top
X2  40.95,74.7 90 top
X3  83.44,69.76 0 top
X4  61.47,67.95 0 top
X5  72.45,63.75 270 top
X6  46.95,69.75 0 top
X7  72.45,65.25 0 top
X8  7.21,54.21 0 top
X9  10.8,42.54 0 top
X10  5.18,64.9 0 top
X11  5.43,74.26 0 top
X12  90.7,31.45 0 top
X13  49.7,31.45 0 top
X14  85.2,31.45 0 top
X15  65.2,30.6 0 top
X16  75.2,26.35 270 top
X17  50.7,31.45 0 top
X18  75.2,27.85 0 top
X19  44.3,54.4 90 top
X20  49.8,49.9 0 top
X21  64.3,48.65 0 top
X22  74.3,45.9 0 top
X23  84.3,49.9 0 top
X24  89.75,49.9 0 top
X25  74.3,44.4 270 top
X26  8.85,15.85 0 top
X27  9.85,15.85 0 top
X28  24.35,15.2 0 top
X29  34.35,12.55 0 top
X30  44.35,15.85 0 top
X31  49.85,15.85 0 top
X32  34.35,11.05 270 top
X33  92.85,16.75 180 top
X34  83.9,5.05 0 top
X35  66.05,16.45 270 top
X36  30.25,70.8 270 top
X37  30.25,69.8 270 top
X38  29.4,55.3 270 top
X39  26.95,45.3 270 top
X40  30.25,35.3 270 top
X41  30.25,29.8 270 top
X42  25.45,45.3 180 top
X43  16.65,31.25 180 top

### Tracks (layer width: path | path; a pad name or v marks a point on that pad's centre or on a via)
GND
  pour Top: 0,0 100,0 100,80 0,80
  pour Bottom: 0,0 100,0 100,80 0,80
N$1
  Top 0.15: X2.1 J1.P$3
N$2
  Top 0.15: X2.2 45.99,69.88 46.8,69.88 X6.1
N$3
  Top 0.15: X6.2 56.06,69.88 56.88,69.88 X4.1
N$4
  Top 0.15: X4.2 65.97,69.88 67.44,69.88 X7.1
N$5
  Top 0.15: X7.2 77.51,69.88 78.81,69.88 X3.1
N$6
  Top 0.15: X5.1 72.47,63.38 72.47,65.16 X7.3
N$7
  Top 0.15: J3.P$3 72.47,59.8 72.47,61.1 X5.2
N$8
  Top 0.15: X1.2 88.89,69.88 88.08,69.88 X3.2
N$9
  Top 0.15: J2.P$3 94.09,63.7 94.09,64.67 X1.1
N$11
  Top 0.15: J4.P$3 45.66,26.32 45.66,27.3 X13.2
N$12
  Top 0.15: X13.1 49.73,31.52 50.7,31.52 X17.1
N$13
  Top 0.15: X17.2 59.8,31.52 60.61,31.52 X15.1
N$14
  Top 0.15: X15.2 69.71,31.52 71.17,31.52 X18.1
N$15
  Top 0.15: X14.1 80.6,31.52 79.3,31.52 X18.2
N$16
  Top 0.15: X16.1 75.24,26 75.24,27.79 X18.3
N$17
  Top 0.15: J6.P$3 75.24,22.43 75.24,23.73 X16.2
N$18
  Top 0.15: X14.2 89.7,31.52 90.67,31.52 X12.2
N$19
  Top 0.15: J5.P$3 94.9,26.32 94.9,27.3 X12.1
N$20
  Top 0.15: J7.P$3 44.36,55.41 44.36,54.44 X19.2
N$21
  Top 0.15: X19.1 48.91,49.89 49.73,49.89 X20.1
N$22
  Top 0.15: X20.2 58.83,49.89 59.8,49.89 X21.1
N$23
  Top 0.15: X21.2 68.9,49.89 70.2,49.89 X22.1
N$24
  Top 0.15: X23.1 79.79,49.89 78.33,49.89 X22.2
N$25
  Top 0.15: X25.1 74.42,44.04 74.42,45.83 X22.3
N$26
  Top 0.15: J9.P$3 74.42,40.46 74.42,41.76 X25.2
N$27
  Top 0.15: X23.2 88.89,49.89 89.7,49.89 X24.2
N$28
  Top 0.15: X24.1 J8.P$3
N$29
  Top 0.15: X26.2 5.04,12.03 5.04,11.05 J10.P$3
N$30
  Top 0.15: X26.1 8.94,15.93 9.75,15.93 X27.1
N$31
  Top 0.15: X27.2 18.85,15.93 19.82,15.93 X28.1
N$32
  Top 0.15: X28.2 28.93,15.93 30.23,15.93 X29.1
N$33
  Top 0.15: X30.1 39.81,15.93 38.35,15.93 X29.2
N$34
  Top 0.15: X32.1 34.45,10.56 34.45,12.51 X29.3
N$35
  Top 0.15: J12.P$3 34.45,7.15 34.45,8.45 X32.2
N$36
  Top 0.15: X30.2 48.91,15.93 49.73,15.93 X31.2
N$37
  Top 0.15: X31.1 53.79,12.03 53.79,11.05 J11.P$3
N$38
  Top 0.15: X36.2 26.49,74.42 25.68,74.42 J13.P$3
N$39
  Top 0.15: X37.1 30.23,69.88 30.23,70.69 X36.1
N$40
  Top 0.15: X38.1 30.23,59.8 30.23,60.77 X37.2
N$41
  Top 0.15: X38.2 30.23,50.7 30.23,49.4 X39.1
N$42
  Top 0.15: X40.1 30.23,39.81 30.23,41.27 X39.2
N$43
  Top 0.15: X42.1 25.51,45.34 26.81,45.34 X39.3
N$44
  Top 0.15: X42.2 22.43,45.34 21.45,45.34 J15.P$3
N$45
  Top 0.15: X41.2 30.23,29.9 30.23,30.71 X40.2
N$46
  Top 0.15: X41.1 26.49,26.16 25.68,26.16 J14.P$3

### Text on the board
tNames: MICROSTRIP 25 OHM | MICROSTRIP 100 OHM | MICROSTRIP SQRT(25*50) OHM | MICROSTRIP 50 OHM | MICROSTRIP SQRT(50*100) OHM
